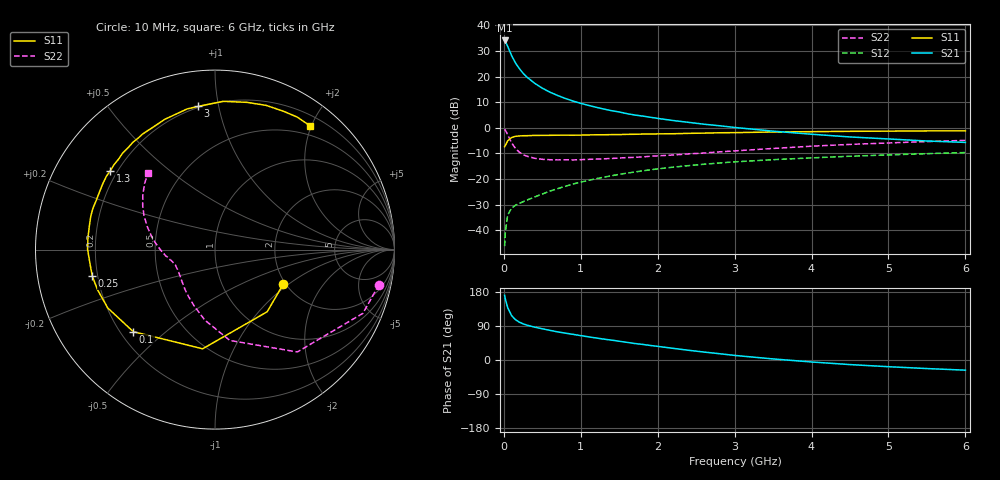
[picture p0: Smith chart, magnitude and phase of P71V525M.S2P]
! SIEMENS Small Signal Semiconductors
! BFP196
! Si NPN RF Bipolar Junction Transistor in SOT143
! VCE = 1.5 V  IC = 25 mA
! Common Emitter S-Parameters:  May  1996
# GHz  S  MA  R  50
!  f  S11  S21  S12  S22
! GHz  MAG  ANG  MAG  ANG  MAG  ANG  MAG  ANG
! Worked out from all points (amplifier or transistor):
!   36 points, 10 MHz to 6 GHz, reference 50 ohm
!   highest |S21| = 34.1 dB at 10 MHz (marker M1)
!   |S21| within 3 dB of that: start of sweep to 60.01 MHz
!   unconditionally stable (mu >= 1): 573.8 MHz to 4.232 GHz
!   at 250 MHz: K = 0.68, MSG = 25.1 dB, |S12| = -28.8 dB
!   at 1.4 GHz: K = 1.11, MAG = 10.7 dB, |S12| = -18.7 dB
!   at 6 GHz: K = 0.99, MSG = 2.0 dB, |S12| = -9.7 dB
!   S11 on the Smith chart (normalised r, x): 10 MHz: 1.94, -0.92; 100 MHz: 0.25, -0.39; 250 MHz: 0.18, -0.10; 1.3 GHz: 0.17, +0.33; 3 GHz: 0.19, +0.87; 6 GHz: 0.35, +1.97
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0.01  0.4262 -27.0  50.51 170.6  0.0049 80.3  0.9339 -12.1
0.02  0.4521 -50.0  48.02 160.2  0.0095 72.5  0.8975 -23.3
0.05  0.557 -97.1  38.79 138.2  0.0198 55.6  0.7319 -51.2
0.1  0.6453 -134.9  25.83 117.3  0.027 44.1  0.5129 -80.7
0.15  0.6802 -151.4  18.54 106.6  0.0307 41.5  0.3973 -98.1
0.2  0.6917 -161.1  14.37 100.0  0.0333 41.6  0.3356 -110.1
0.25  0.6993 -167.8  11.59 95.4  0.0361 43.3  0.2988 -119.9
0.3  0.7003 -172.7  9.736 92.0  0.0388 45.4  0.2788 -126.6
0.4  0.71 179.8  7.395 86.7  0.0446 48.5  0.254 -136.8
0.5  0.7109 174.6  5.923 82.4  0.0511 51.7  0.2423 -144.0
0.6  0.7124 169.3  4.947 78.2  0.0581 53.5  0.2381 -148.8
0.7  0.7167 164.8  4.259 74.1  0.065 54.4  0.2364 -152.5
0.9  0.7161 157.4  3.317 67.7  0.0801 55.0  0.2359 -158.0
1.1  0.7246 149.8  2.734 61.1  0.0942 54.7  0.242 -161.6
1.3  0.7302 142.9  2.318 55.1  0.1088 53.4  0.2481 -165.0
1.7  0.7466 130.2  1.776 43.6  0.137 49.7  0.2653 -170.7
2.2  0.7646 116.7  1.385 30.8  0.1704 43.6  0.2943 -177.4
3  0.8035 96.7  1.015 12.1  0.2163 32.8  0.3538 169.7
3.5  0.8272 86.9  0.859 2.8  0.2386 26.4  0.3949 161.9
4.5  0.8525 70.5  0.662 -12.1  0.2783 14.7  0.4736 148.3
5.5  0.8689 58.2  0.552 -22.6  0.3126 3.9  0.5381 136.8
6  0.8695 52.6  0.518 -26.8  0.3291 -2.0  0.5677 131.0
